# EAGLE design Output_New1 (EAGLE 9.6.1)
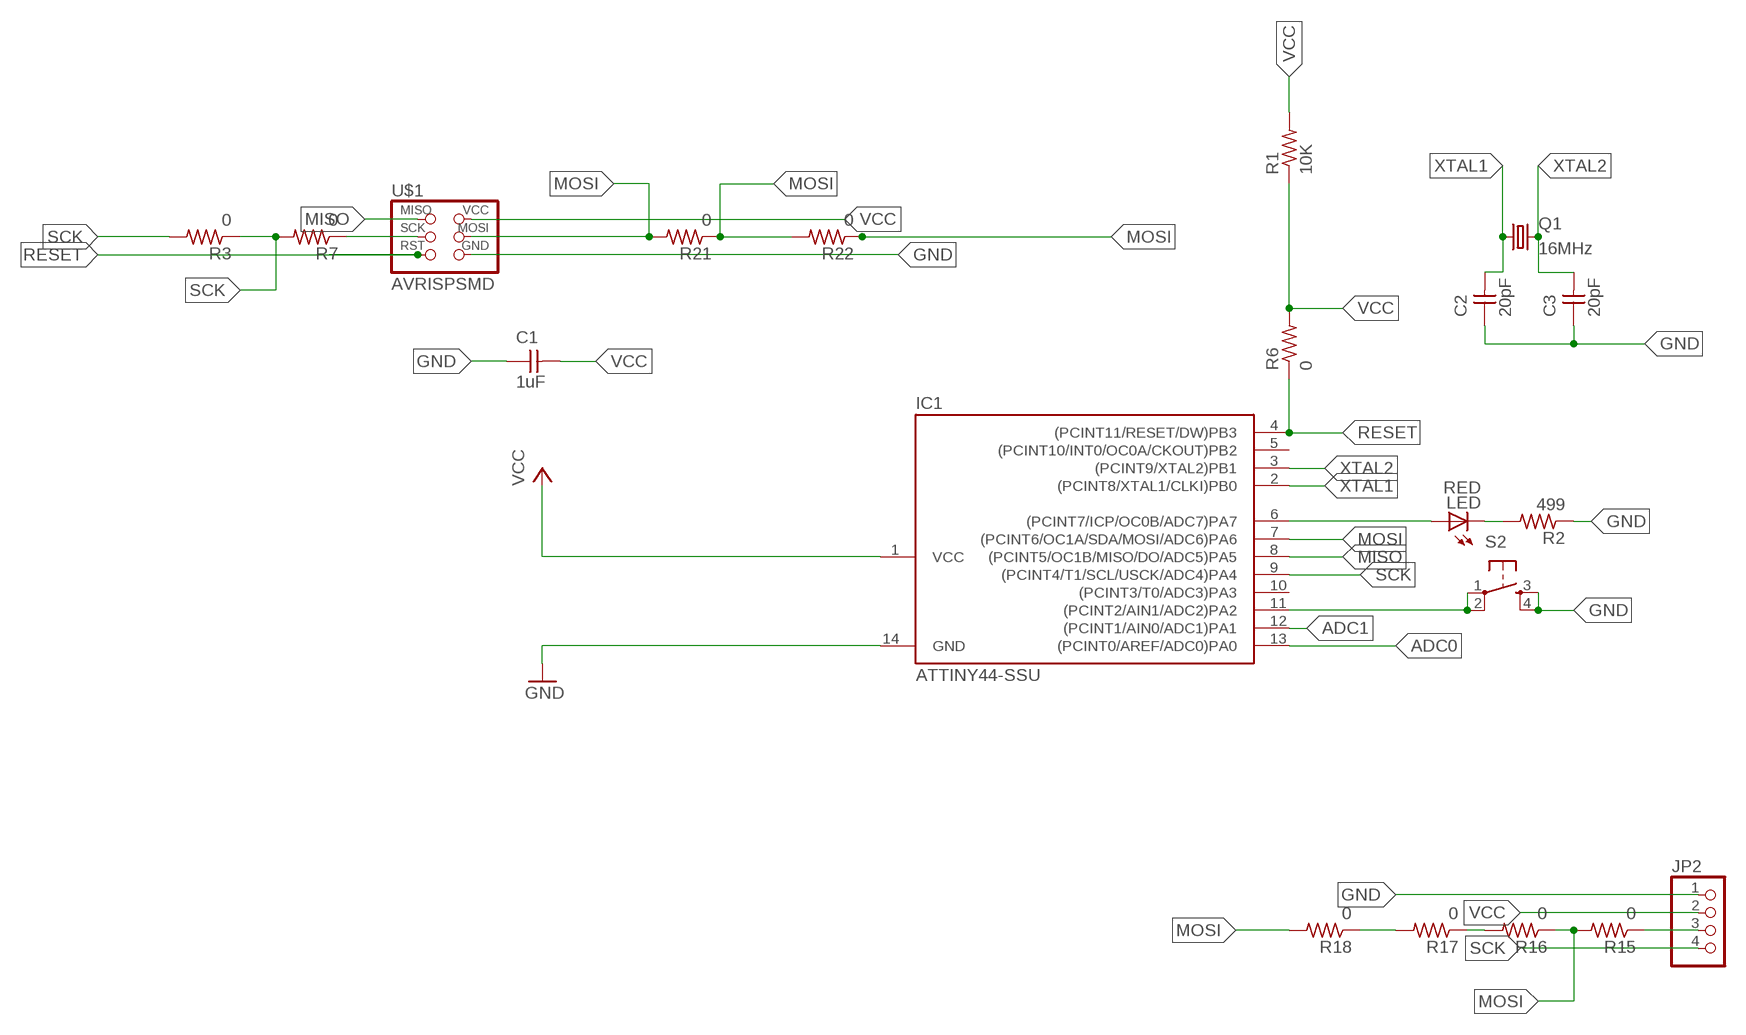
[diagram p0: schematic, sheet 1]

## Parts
C1  1uF  UNPOLARIZED_CAPACITOR1206  [1206]
C2  20pF  UNPOLARIZED_CAPACITOR1206  [1206]
C3  20pF  UNPOLARIZED_CAPACITOR1206  [1206]
IC1  ATTINY44-SSU  [SOIC14]
JP2  PINHD-1X4  [1X04]
LED  RED  LED1206  [1206]
Q1  16MHz  CSM-7X-DU  [CSM-7X-DU]
R1  10K  RESISTOR1206  [1206]
R2  499  RESISTOR1206  [1206]
R3  0  RESISTOR1206  [1206]
R6  0  RESISTOR1206  [1206]
R7  0  RESISTOR1206  [1206]
R15  0  RESISTOR1206  [1206]
R16  0  RESISTOR1206  [1206]
R17  0  RESISTOR1206  [1206]
R18  0  RESISTOR1206  [1206]
R21  0  RESISTOR1206  [1206]
R22  0  RESISTOR1206  [1206]
S2  6MM_SWITCH6MM_SWITCH  [6MM_SWITCH]
U$1  AVRISPSMD  [2X03SMD]

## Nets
ADC0: IC1.13((PCINT0/AREF/ADC0)PA0)
ADC1: IC1.12((PCINT1/AIN0/ADC1)PA1)
GND: C1.1 C2.1 C3.1 IC1.14(GND) JP2.1 R2.1 S2.3(S) S2.4(S1) U$1.6(GND)
MISO: IC1.8((PCINT5/OC1B/MISO/DO/ADC5)PA5) U$1.1(MISO)
MOSI: IC1.7((PCINT6/OC1A/SDA/MOSI/ADC6)PA6) JP2.3 R15.1 R15.2 R16.1 R16.2 R17.1 R17.2 R18.1 R18.2 R21.1 R21.2 R22.1 R22.2 U$1.4(MOSI)
N$1: IC1.6((PCINT7/ICP/OC0B/ADC7)PA7) LED.1(A)
N$2: LED.2(C) R2.2
N$11: IC1.11((PCINT2/AIN1/ADC2)PA2) S2.1(P) S2.2(P1)
RESET: IC1.4((PCINT11/RESET/DW)PB3) R6.1 U$1.5(RST)
SCK: IC1.9((PCINT4/T1/SCL/USCK/ADC4)PA4) JP2.4 R3.1 R3.2 R7.1 R7.2 U$1.3(SCK)
VCC: C1.2 IC1.1(VCC) JP2.2 R1.1 R1.2 R6.2 U$1.2(VCC)
XTAL1: C2.2 IC1.2((PCINT8/XTAL1/CLKI)PB0) Q1.1
XTAL2: C3.2 IC1.3((PCINT9/XTAL2)PB1) Q1.2
Unconnected: IC1.5((PCINT10/INT0/OC0A/CKOUT)PB2) IC1.10((PCINT3/T0/ADC3)PA3)

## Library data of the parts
C1-C3 = FAB_Hello:UNPOLARIZED_CAPACITOR: unpolarized_capacitor
IC1 = FAB_Hello:ATTINY44
JP2 = pinhead:PINHD-1X4: PIN HEADER
LED = FAB_Hello:LED
Q1 = FAB_Hello:CSM-7X-DU: SMD CRYSTAL; OC_FARNELL: unknown; OC_NEWARK: unknown
R1-R3 R6 R7 R15-R18 R21 R22 = FAB_Hello:RESISTOR
S2 = fab:6MM_SWITCH: OMRON SWITCH
U$1 = FAB_Hello:AVRISP

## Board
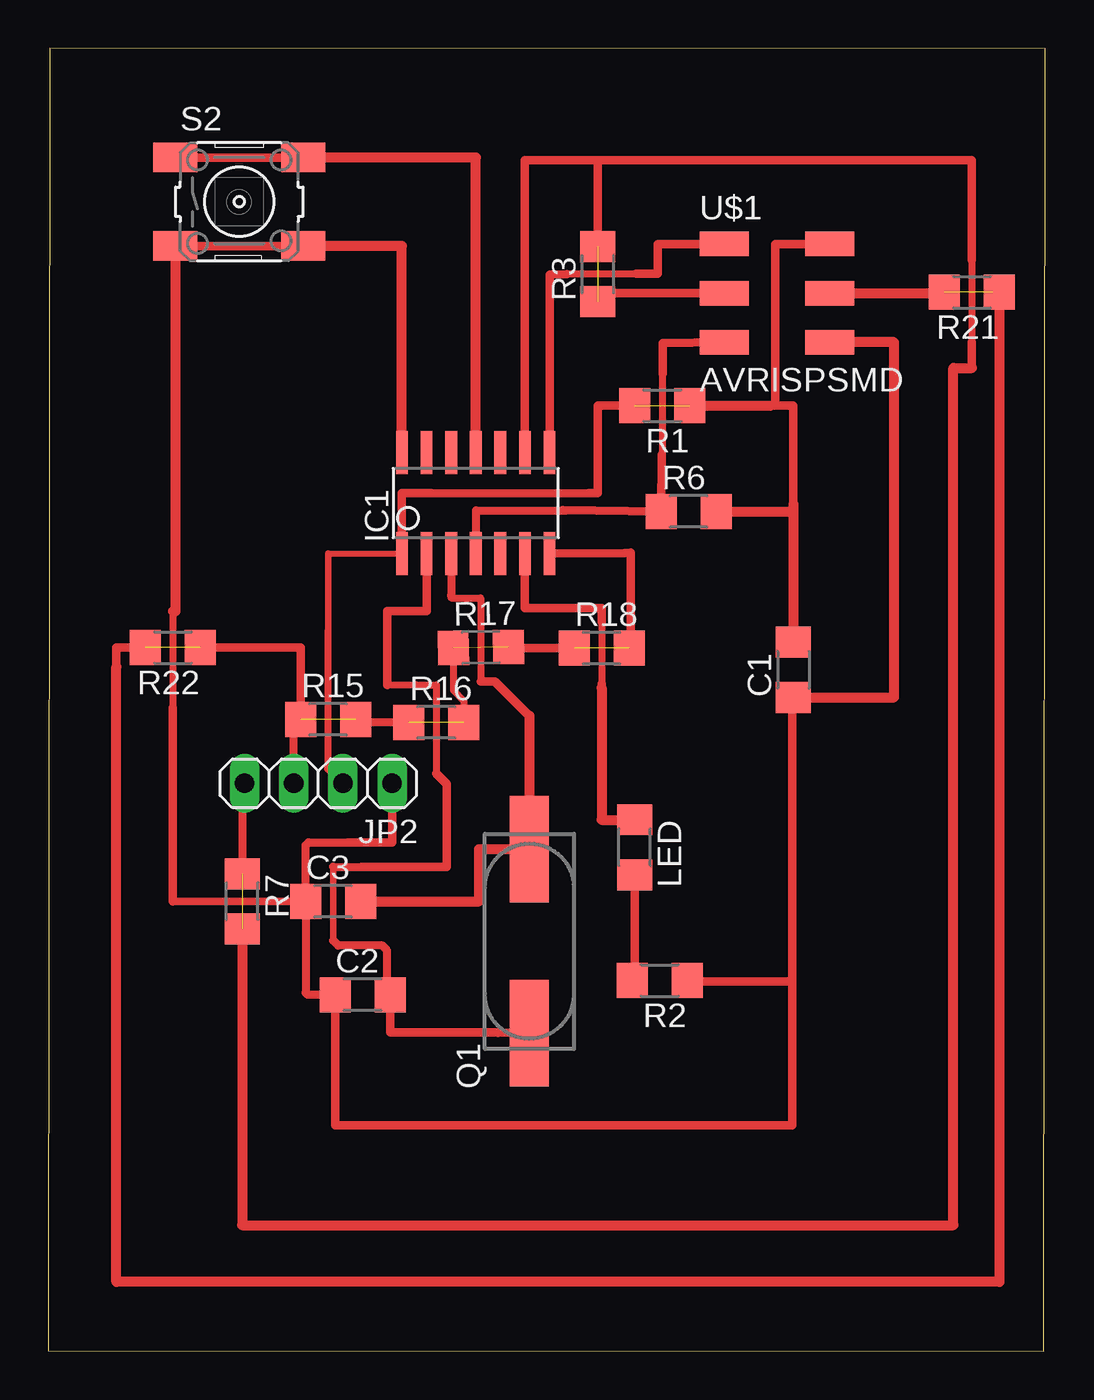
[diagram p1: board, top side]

Size 51.49 x 67.31 mm. Coordinates in mm from the lower left corner, seen from the top.
Outline: 0,0.03 51.41,0 51.49,67.28 0.08,67.31 0,0.03
Copper layers (1*16): Top 0.035mm / dielectric 1.5mm / Bottom 0.035mm
Design rules "default *": minimum track width 6mil, minimum drill 0.35mm, track to track 17mil, track to pad 17mil, pad to pad 17mil, via to via 17mil, smd to smd 17mil, copper to edge 40mil, drill to drill 6mil, minimum pad ring 10mil, minimum via ring 8mil, stop-mask expansion 4mil, vias tented up to drill 0mil, thermal gap 17mil

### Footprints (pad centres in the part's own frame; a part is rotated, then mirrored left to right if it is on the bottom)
1206 = smd 1.6 x 1.803: 1 -1.422,0; 2 1.422,0
SOIC14 = smd 0.61 x 2.21: 1 -3.81,-2.603; 2 -2.54,-2.603; 3 -1.27,-2.603; 4 0,-2.603; 5 1.27,-2.603; 6 2.54,-2.603; 7 3.81,-2.603; 8 3.81,2.603; 9 2.54,2.603; 10 1.27,2.603; 11 0,2.603; 12 -1.27,2.603; 13 -2.54,2.603; 14 -3.81,2.603
1X04 = drill 1.016 long: 1 -3.81,0; 2 -1.27,0; 3 1.27,0; 4 3.81,0
CSM-7X-DU = smd 5.5 x 2: 1 -4.75,0; 2 4.75,0
6MM_SWITCH = smd 2.286 x 1.524: 1 -3.302,2.286; 2 3.302,2.286; 3 -3.302,-2.286; 4 3.302,-2.286
2X03SMD = smd 2.54 x 1.27: 1 -2.54,2.54; 2 2.92,2.54; 3 -2.54,0; 4 2.92,0; 5 -2.54,-2.54; 6 2.92,-2.54

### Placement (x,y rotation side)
C1  38.48,35.2 90 top
C2  16.23,18.41 0 top
C3  14.71,23.24 0 top
IC1  22.07,43.81 0 top
JP2  13.94,29.34 180 top
LED  30.28,26.04 270 top
Q1  24.84,21.18 90 top
R1  31.7,48.84 180 top
R2  31.57,19.15 180 top
R3  28.37,55.65 90 top
R6  33.07,43.38 0 top
R7  10.01,23.24 270 top
R15  14.45,32.64 0 top
R16  20.04,32.49 0 top
R17  22.34,36.36 1 top
R18  28.58,36.32 0 top
R21  47.7,54.71 180 top
R22  6.43,36.35 180 top
S2  9.86,59.39 0 top
U$1  37.44,54.66 0 top

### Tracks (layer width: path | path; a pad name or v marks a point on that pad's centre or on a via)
GND
  Top 0.356: 6.43,38.23 6.43,33.25
  Top 0.381: R2.1 32.78,18.94 32.64,18.8 | 6.43,23.24 C3.1
  Top 0.406: 15.47,26.29 13.44,26.29 13.28,26.14 C3.1 13.28,18.52 13.39,18.41 C2.1
  Top 0.432: C2.1 14.81,11.66 38.43,11.66 38.43,19.1 | 33.17,19.15 R2.1 | 6.43,33.25 6.43,23.24 | 15.47,26.29 17.75,26.29 JP2.1 | 13.46,57.1 S2.4 S2.3 | 38.43,19.1 32.78,19.1 32.78,18.94 | C1.1 38.43,33.78 38.43,19.1
  Top 0.508: S2.3 6.55,38.23 6.43,38.23 | IC1.14 18.26,57.1 13.46,57.1 | C1.1 43.69,33.78 43.69,52.12 U$1.6
MISO
  Top 0.356: 26.77,55.63 26.77,55.66 30.35,55.66
  Top 0.432: IC1.8 25.88,55.63 26.77,55.63 | 30.35,55.66 31.47,55.66 31.47,57.2 U$1.1
MOSI  (6 unrouted)
  Top 0.33: 12.67,29.74 JP2.3
  Top 0.356: R17.1 20.91,34.16 21.46,33.58 R16.2 | R17.2 23.85,36.38
  Top 0.406: JP2.3 12.67,32.28 R15.1 | 25.98,41.11 IC1.7 | R16.1 16.03,32.49 R15.2
  Top 0.432: R22.1 13.03,36.35 R15.1 | IC1.7 29.77,41.25 30.07,41.25 30.07,36.32 R18.2 | R21.1 48.77,54.71 | R22.2 3.51,36.35 3.51,35.36 | R18.1 23.76,36.32 R17.2
  Top 0.508: R21.1 49.12,3.58 3.51,3.58 3.51,35.36 | U$1.4 46.28,54.66 R21.2
N$1
  Top 0.356: 28.57,37.67 28.57,34.49
  Top 0.432: IC1.6 24.61,38.41 28.57,38.41 28.57,37.67 | 28.57,34.49 28.57,34.27
  Top 0.508: 28.57,34.27 28.57,27.46 LED.1
N$2
  Top 0.432: LED.2 30.28,19.15 R2.2
N$11
  Top 0.432: 13.46,61.67 S2.2 S2.1
  Top 0.508: IC1.11 22.07,61.67 13.46,61.67
RESET
  Top 0.356: 31.72,50.49 31.7,50.47 31.7,46.33 31.68,46.33
  Top 0.406: 26.77,43.43 26.54,43.43 22.07,43.43 IC1.4
  Top 0.432: R6.1 31.29,43.38 | R6.1 26.56,43.45 26.54,43.43 | U$1.5 31.74,52.07 31.72,50.49 | 31.68,46.33 R6.1
SCK  (2 unrouted)
  Top 0.356: 47.7,56.36 47.7,52.12
  Top 0.406: IC1.9 24.61,48.64 | JP2.4 10.01,29.21 R7.1 | 9.65,21.46 R7.2
  Top 0.432: IC1.9 24.61,61.54 28.37,61.54 | 28.37,61.54 47.7,61.54 47.7,56.36 | 47.7,50.8 47.7,52.12 | R7.2 9.73,21.82 | R3.2 28.37,61.54 | U$1.3 28.8,54.66 R3.1
  Top 0.508: R7.2 10.01,6.5 46.74,6.5 46.74,50.8 47.7,50.8
VCC  (1 unrouted)
  Top 0.305: 14.45,41.21 IC1.1
  Top 0.33: 14.45,37.21 14.45,41.21
  Top 0.356: 14.45,30.1 14.45,37.21
  Top 0.406: 19.79,44.32 27.91,44.32 | JP2.2 14.45,30.1
  Top 0.432: IC1.1 18.26,44.32 19.79,44.32 | 27.91,44.32 28.37,44.32 28.37,48.84 R1.2 | 38.28,43.38 38.48,43.38 | 38.48,43.38 C1.2 | 37.26,48.84 37.54,48.84 | 37.54,48.84 38.48,48.84 38.48,43.76 38.48,43.38 | U$1.2 37.54,57.2 37.54,48.84
  Top 0.508: R6.2 38.28,43.38 | 38.48,43.76 C1.2 | R1.1 37.26,48.84
XTAL1
  Top 0.33: 14.71,21.21 14.71,25.02 | 17.5,34.42 19.02,34.42
  Top 0.356: 19.02,34.42 20.04,34.42 20.04,29.84
  Top 0.406: Q1.1 23.22,16.43 23.19,16.46 | C2.2 17.5,18.57 17.5,20.7 17.25,20.95 14.96,20.95 14.71,21.21 | 14.71,25.02 16.18,25.02
  Top 0.432: 16.18,25.02 20.57,25.02 20.57,29.31 20.04,29.84 | C2.2 17.65,16.46 23.19,16.46 | 17.5,34.42 17.5,38.23 19.53,38.23 IC1.2
XTAL2
  Top 0.356: 20.8,39.06 20.8,38.91 22.33,38.91 22.33,34.59
  Top 0.406: IC1.3 20.8,39.06
  Top 0.432: 24.84,32.82 23.06,34.59 22.33,34.59
  Top 0.508: C3.2 22.25,23.24 22.25,25.93 Q1.2 24.84,32.82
